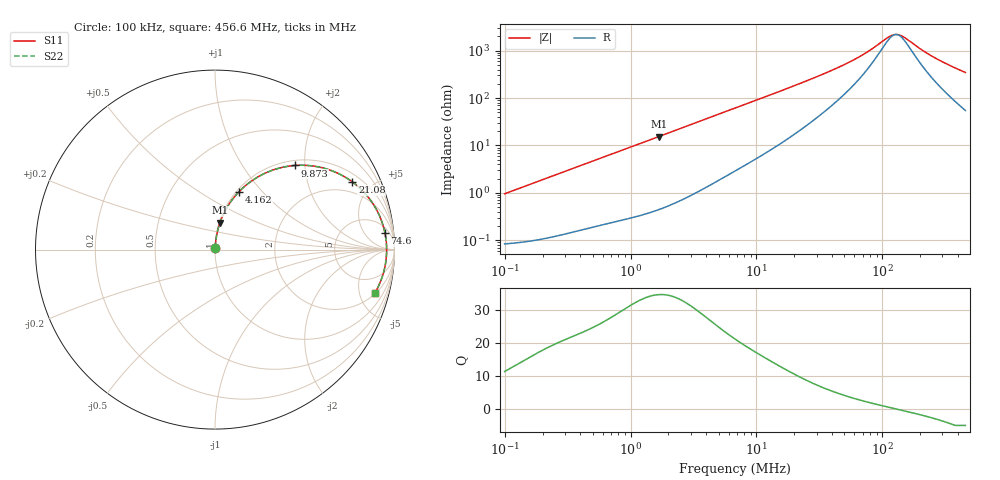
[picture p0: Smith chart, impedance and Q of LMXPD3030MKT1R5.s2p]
! LMXPD3030MKT1R5  S-PARAMETER MODEL  ( General Type )
! Model Generated by TAIYO YUDEN Corporation (http://www.ty-top.com)
! Version 1.0
! TAIYO YUDEN Control No. 191023NI43SB-FBB
! Copyright(c) 2019 TAIYO YUDEN CO.,LTD. All Rights Reserved.
! Product Description (link to TY-COMPAS)
! https://ds.yuden.co.jp/TYCOMPAS/or/detail?pn=LMXPD3030MKT1R5N&u=M
! Products Name : Inductors
! Characteristics :
!  Inductance : 1.5 uH , SRF(min) : 92 MHz , DC Resistance(max) : 0.09 Ohm
!  Rated Current : Saturation :2100 mA , Temp Rise : 1400 mA
!  Case Size : 3.0 x 3.0 / 0.118 x 0.118 [mm/inch] , Thickness : 1.2 / 0.047 [mm/inch]
!  (Conditions: Temperature = 25 degC , DC Bias Current/Voltage = 0A / 0V)
! External Node Assignments :
!  1  o---GGG---o  2
! GND o---------o GND
! Frequency Range : 0.1MHz  -  456.598367MHz  [ 402 STEP ]
# MHz S RI R 50
! Freq[MHz].  S11 Real  S11 Imag  S21 Real  S21 Imag  S12 Real  S12 Imag  S22 Real  S22 Imag
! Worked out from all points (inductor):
!   401 points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, 100 kHz to 456.6 MHz, reference 50 ohm
!   read as one part in series: L = 1.52 uH near 104.3 kHz
!   highest Q = 34.7 at 1.682 MHz (marker M1), where L = 1.46 uH
!   self-resonance near 128.7 MHz
!   S11 on the Smith chart (normalised r, x): 100 kHz: 1.00, +0.02; 4.162 MHz: 1.03, +0.76; 9.873 MHz: 1.10, +1.78; 21.08 MHz: 1.38, +3.83; 74.6 MHz: 9, +17; 456.6 MHz: 2.09, -6.84
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0.1  0.000929 0.00952  0.9991 -0.00952  0.9991 -0.00952  0.000929 0.00952
0.410178  0.00313 0.0383  0.9969 -0.0383  0.9969 -0.0383  0.00313 0.0383
0.894291  0.00945 0.0816  0.9906 -0.0816  0.9906 -0.0816  0.00945 0.0816
1.682457  0.0274 0.1495  0.9726 -0.1495  0.9726 -0.1495  0.0274 0.1495
2.789434  0.0676 0.2359  0.9324 -0.2359  0.9324 -0.2359  0.0676 0.2359
4.162401  0.1347 0.3235  0.8653 -0.3235  0.8653 -0.3235  0.1347 0.3235
5.35957  0.2015 0.3808  0.7985 -0.3808  0.7985 -0.3808  0.2015 0.3808
6.901063  0.2901 0.4306  0.7099 -0.4306  0.7099 -0.4306  0.2901 0.4306
9.872934  0.4461 0.4689  0.5539 -0.4689  0.5539 -0.4689  0.4461 0.4689
14.12461  0.6119 0.4522  0.3881 -0.4522  0.3881 -0.4522  0.6119 0.4522
21.07678  0.7658 0.3769  0.2342 -0.3769  0.2342 -0.3769  0.7658 0.3769
27.71655  0.8396 0.309  0.1604 -0.309  0.1604 -0.309  0.8396 0.309
47.93016  0.9211 0.1777  0.0789 -0.1777  0.0789 -0.1777  0.9211 0.1777
74.59925  0.9474 0.0906  0.0526 -0.0906  0.0526 -0.0906  0.9474 0.0906
113.6871  0.9559 0.0199  0.0441 -0.0199  0.0441 -0.0199  0.9559 0.0199
126.3151  0.9564 0.00302  0.0436 -0.00302  0.0436 -0.00302  0.9564 0.00302
140.3458  0.9562 -0.0138  0.0438 0.0138  0.0438 0.0138  0.9562 -0.0138
155.935  0.9554 -0.0308  0.0446 0.0308  0.0446 0.0308  0.9554 -0.0308
209.4245  0.9497 -0.0803  0.0503 0.0803  0.0503 0.0803  0.9497 -0.0803
253.1436  0.9425 -0.1148  0.0575 0.1148  0.0575 0.1148  0.9425 -0.1148
339.9779  0.9235 -0.1745  0.0765 0.1745  0.0765 0.1745  0.9235 -0.1745
456.5984  0.8902 -0.2428  0.1098 0.2428  0.1098 0.2428  0.8902 -0.2428
